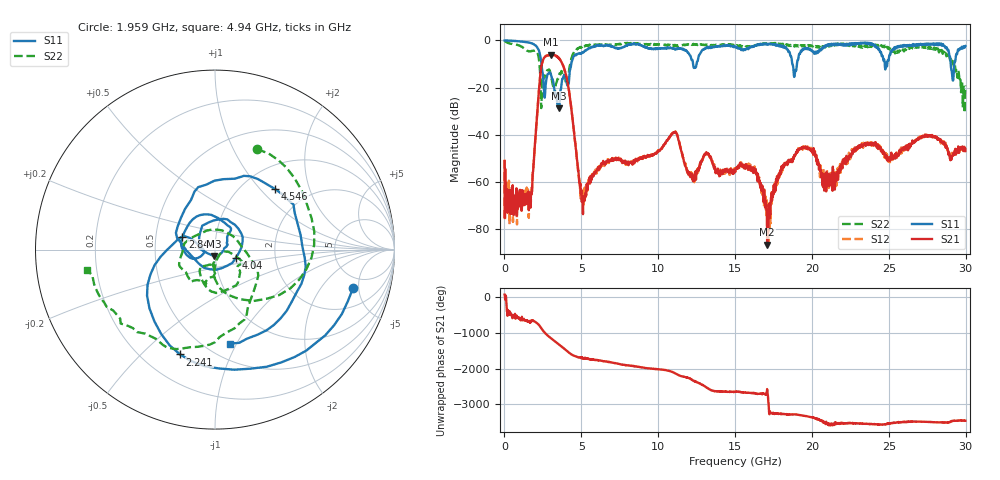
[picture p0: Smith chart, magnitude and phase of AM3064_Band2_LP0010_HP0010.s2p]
# Hz S DB R 50.0
!freq dBS11 angS11 dBS21 angS21 dBS12 angS12 dBS22 angS22
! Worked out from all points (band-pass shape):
!   1600 points, 10 MHz to 29.98 GHz, reference 50 ohm
!   highest |S21| = -6.11 dB at 3.046 GHz (marker M1); lowest = -86.7 dB at 17.09 GHz (marker M2)
!   |S21| within 3 dB of the highest: 2.469 GHz to 3.702 GHz (1.233 GHz wide, 40 % of centre)
!   lowest |S11| = -28.9 dB at 3.553 GHz (marker M3), VSWR 1.07, Z = 49.5 - j3.54 ohm
!   |S11| at or under -10 dB: 2.404 GHz to 4.345 GHz (1.94 GHz wide, 57.5 % of centre); 18.73 GHz to 19.02 GHz (289.4 MHz wide, 1.53 % of centre); 29.03 GHz to 29.26 GHz (230.4 MHz wide, 0.791 % of centre)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
!   |S22| runs from -30.7 to -0.2 dB; largest |S21 - S12| = 0.014
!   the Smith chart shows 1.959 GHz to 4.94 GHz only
!   S11 on the Smith chart (normalised r, x): 1.959 GHz: 3.69, -4.34; 2.241 GHz: 0.35, -0.66; 2.84 GHz: 0.69, +0.10; 4.04 GHz: 1.25, -0.12; 4.546 GHz: 1.39, +1.21; 4.94 GHz: 0.65, -0.94
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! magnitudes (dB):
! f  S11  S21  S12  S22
! 10 MHz  0.0  -51.2  -50.6  -0.2
! 1.566 GHz  -0.9  -64.1  -69.3  -4.6
! 1.959 GHz  -2.0  -46.0  -46.1  -4.3
! 2.241 GHz  -4.2  -21.4  -21.4  -8.0
! 2.84 GHz  -14.2  -6.4  -6.3  -12.6
! 3.046 GHz  -15.1  -6.1  -6.1  -15.7
! 3.553 GHz  -28.9  -7.8  -7.7  -14.7
! 4.04 GHz  -18.1  -15.8  -15.7  -18.9
! 4.546 GHz  -6.5  -40.1  -39.9  -4.8
! 4.94 GHz  -5.5  -60.7  -65.8  -2.8
! 5.015 GHz  -5.6  -65.2  -64.2  -3.0
! 10 GHz  -3.5  -47.1  -46.6  -1.8
! 15 GHz  -2.6  -55.9  -55.7  -1.9
! 16.28 GHz  -2.2  -55.0  -55.8  -2.2
! 17.09 GHz  -1.5  -86.7  -72.0  -1.6
! 18.15 GHz  -2.7  -53.9  -53.5  -2.1
! 19.99 GHz  -4.2  -46.7  -46.8  -2.2
! 20.83 GHz  -2.9  -59.0  -64.5  -2.4
! 25 GHz  -8.0  -50.2  -51.1  -3.0
! 28.56 GHz  -2.3  -43.9  -44.1  -4.8
! 29.18 GHz  -17.1  -48.4  -48.5  -9.0
! 29.98 GHz  -2.4  -47.0  -47.8  -19.2
